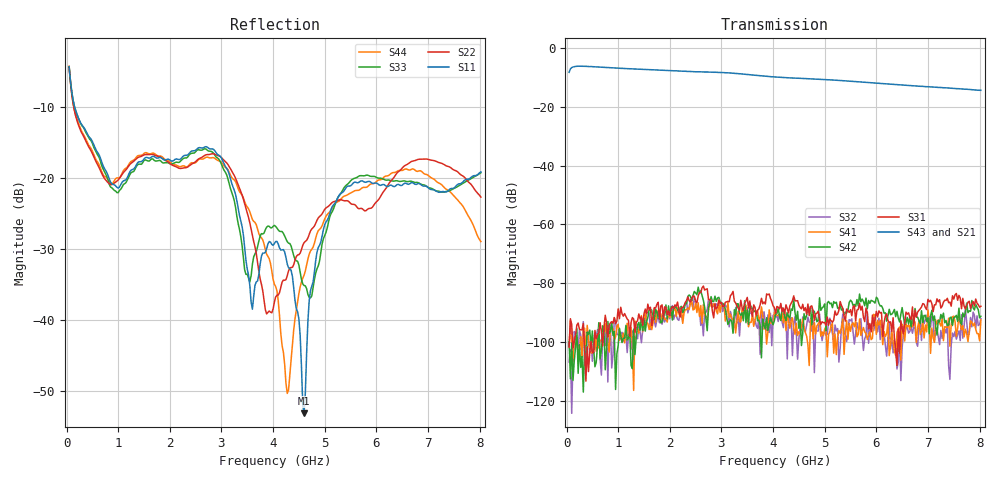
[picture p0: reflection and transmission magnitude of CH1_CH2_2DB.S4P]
!Agilent Technologies,E5071C,MY46316741,A.11.02
!Date: Thu May 28 14:26:02 2026
!Data & Calibration Information:
!1:CH1 INPUT 2:CH1 OUTPUT 3:CH2 INPUT 4:CH2 OUTPUT
!Freq	S11:SOLT4(ON)	S12:SOLT4(ON)	S13:SOLT4(ON)	S14:SOLT4(ON)
!	S21:SOLT4(ON)	S22:SOLT4(ON)	S23:SOLT4(ON)	S24:SOLT4(ON)
!	S31:SOLT4(ON)	S32:SOLT4(ON)	S33:SOLT4(ON)	S34:SOLT4(ON)
!	S41:SOLT4(ON)	S42:SOLT4(ON)	S43:SOLT4(ON)	S44:SOLT4(ON)
!PortZ  Port1:50+j0  Port2:50+j0  Port3:50+j0  Port4:50+j0
!Above PortZ is port z conversion or system Z0 setting when saving the data.
!When reading, reference impedance value at option line is always used.
# Hz S dB R 50
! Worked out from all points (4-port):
!   320 points, 50 MHz to 8.025 GHz, reference 50 ohm
!   strongest paths, dB at 50 MHz, 2.05 GHz, 4.05 GHz, 6.05 GHz, 8.025 GHz:
!     S43: -8.2, -7.7, -9.8, -12.0, -14.4
!     S21: -8.4, -7.8, -9.9, -12.0, -14.4
!     S31: -101.8, -88.0, -90.3, -89.4, -87.9
!     S42: -99.9, -92.6, -90.5, -86.9, -91.3
!     S41: -101.3, -89.9, -89.7, -94.3, -92.5
!     S32: -106.8, -87.6, -91.6, -92.0, -92.1
!   lowest |S11| = -53.1 dB at 4.6 GHz (marker M1), VSWR 1.00, Z = 49.9 + j0.204 ohm
!   |S11| at or under -10 dB: 159.1 MHz to end of sweep
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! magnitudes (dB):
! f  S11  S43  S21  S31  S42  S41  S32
! 50 MHz  -4.3  -8.2  -8.4  -101.8  -99.9  -101.3  -106.8
! 3 GHz  -17.1  -8.3  -8.4  -86.6  -86.8  -87.4  -86.8
! 3.6 GHz  -38.4  -9.1  -9.2  -91.3  -89.0  -90.7  -90.9
! 4.275 GHz  -32.1  -10.1  -10.2  -88.7  -90.0  -90.0  -105.8
! 4.6 GHz  -53.1  -10.3  -10.4  -89.4  -90.4  -95.1  -95.4
! 5.3 GHz  -22.2  -11.0  -11.1  -86.3  -87.6  -97.1  -102.2
! 8.025 GHz  -19.1  -14.4  -14.4  -87.9  -91.3  -92.5  -92.1
